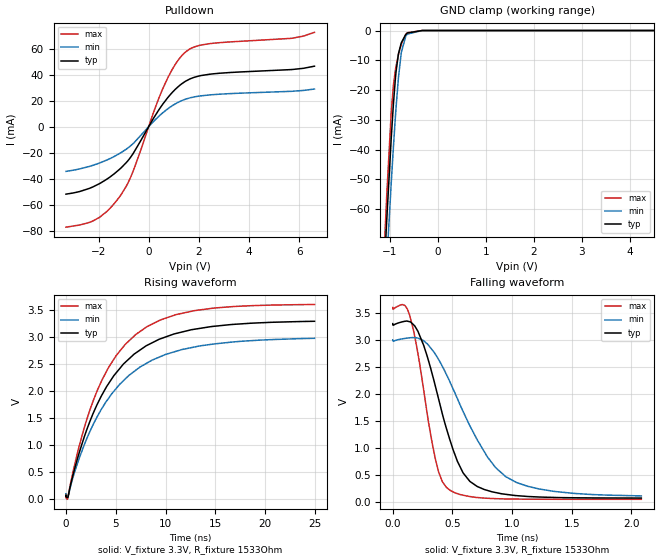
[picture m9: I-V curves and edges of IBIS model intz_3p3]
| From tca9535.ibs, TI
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|   intz_3p3 Model
[Model]   intz_3p3
Model_type   Open_sink
Polarity   Non-Inverting
Vmeas = 1.65
Vref = 3.3
Cref = 100pF
Rref = 1533
|   typ   min   max
|   (nom PVT)   (fast PVT)   (slow PVT)
C_comp   1.340e-12   1.280e-12   1.472e-12
| Where nom  PVT is Nominal Process, 3.3V, 27C
|   Fast PVT is Strong Process,  3.6V, -40C
|   Slow PVT is Weak Process,   3V, 100C
[Voltage Range]   3.3   3   3.6
|Junction Temperature
[Temperature Range]   27   100   -40
[Pullup Reference]   3.3   3   3.6
[Pulldown Reference]   0   0   0
[Power Clamp Reference]   3.3   3   3.6
[GND Clamp Reference]   0   0   0
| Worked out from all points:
|   slope of the pulldown table from 0 to 0.495 V, typ, clamps not added: 32.1 ohm
|   GND clamp passes 1 mA (typ) near -0.65 V on its own axis
|   falling waveform, V_fixture 3.3V, R_fixture 1533Ohm: 20-80 % time 255ps typ, 408ps min, 162ps max; typ from 3.3 V to 0.065 V
|   rising waveform, V_fixture 3.3V, R_fixture 1533Ohm: 20-80 % time 5.53ns typ, 5.94ns min, 5.08ns max; typ from 0.062 V to 3.29 V
[Pulldown]
|   Voltage   I(typ)   I(min)   I(max)
-3.3V     -51.89mA   -34.4mA    -77.26mA
-2.379V   -47.56mA   -30.65mA   -73.7mA
-1.97V    -43.9mA    -28.04mA   -69.8mA
-1.536V   -38.59mA   -24.48mA   -62.62mA
-1.1V     -31.65mA   -19.92mA   -52.2mA
-643.5mV  -21.27mA   -13.39mA   -35.18mA
564.3mV   17.44mA    10.72mA    29.44mA
1.056V    28.63mA    17.47mA    47.82mA
1.47V     34.92mA    21.11mA    57.44mA
2.436V    40.28mA    24.37mA    63.77mA
5.66V     43.8mA     27.11mA    67.8mA
6.6V      46.44mA    28.87mA    72.45mA
[GND Clamp]
|   Voltage   I(typ)   I(min)   I(max)
-3.3V     -935.3mA   -881mA     -1.051A
-1.109V   -76.76mA   -90.34mA   -69.57mA
-1.076V   -66.23mA   -80.39mA   -58.14mA
-1.063V   -62.11mA   -76.46mA   -53.7mA
-973.5mV  -35.98mA   -50.99mA   -27.35mA
-927.6mV  -24.41mA   -38.83mA   -18.23mA
-873mV    -13.74mA   -25.72mA   -11.89mA
-822mV    -7.679mA   -15.52mA   -7.968mA
-765mV    -4.176mA   -7.526mA   -4.647mA
-639mV    -823.3uA   -1.195mA   -739.2uA
-330mV    -858.1nA   -3.249uA   -135.8nA
6.6V      0A         0A         0A
[POWER Clamp]
|   Voltage   I(typ)   I(min)   I(max)
-3.3V     0A         0A         0A
0V        0A         0A         0A
6.6V      0A         0A         0A
[Ramp]
R_load = 1533
|   typ   min   max
dV/dt_r   1.94299/5.59011e-09   1.74586/6.09277e-09   2.13618/5.09873e-09
dV/dt_f   1.94297/2.55938e-10   1.74583/4.10878e-10   2.13619/1.61645e-10
[Falling Waveform]
V_fixture = 3.3V
V_fixture_min = 3V
V_fixture_max = 3.6V
R_fixture = 1533Ohm
|   Time   V(typ)   V(min)   V(max)
0s        3.3V       3V         3.6V
139.4ps   3.337V     3.037V     3.469V
259.6ps   2.892V     2.979V     2.054V
357.7ps   2.131V     2.73V      777.1mV
450.1ps   1.35V      2.354V     260.8mV
541.7ps   745.5mV    1.907V     147.1mV
646ps     374.1mV    1.405V     93.06mV
945.9ps   134.6mV    462.8mV    48.59mV
1.351ns   76.3mV     188.9mV    42.47mV
2.084ns   65.04mV    104.6mV    41.39mV
[Rising Waveform]
V_fixture = 3.3V
V_fixture_min = 3V
V_fixture_max = 3.6V
R_fixture = 1533Ohm
|   Time   V(typ)   V(min)   V(max)
0s        61.71mV    90.25mV    39.67mV
173.4ps   34.48mV    69.59mV    6.721mV
1.391ns   896.4mV    788.2mV    1.025V
2.373ns   1.424V     1.24V      1.633V
3.135ns   1.752V     1.525V     2.005V
5.047ns   2.335V     2.046V     2.654V
7.009ns   2.701V     2.383V     3.042V
9.481ns   2.962V     2.633V     3.31V
12.93ns   3.14V      2.812V     3.483V
24.93ns   3.285V     2.971V     3.595V
